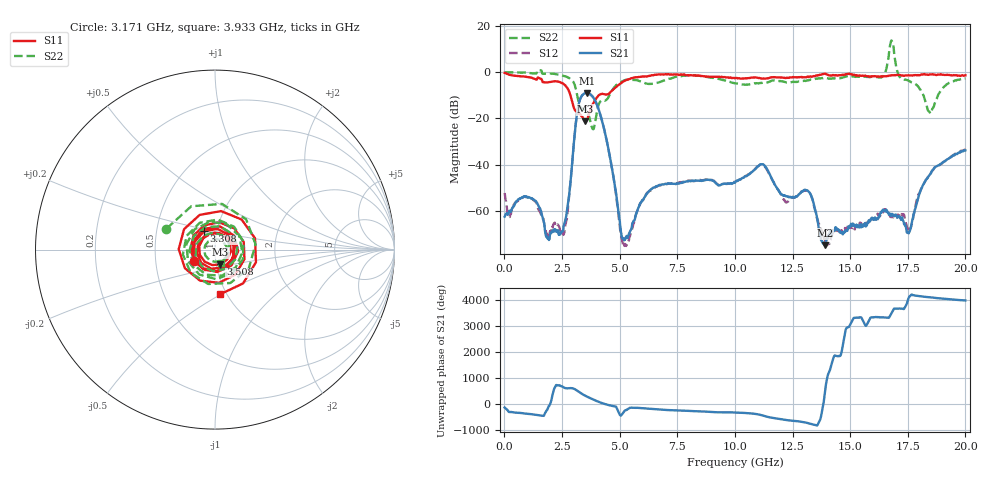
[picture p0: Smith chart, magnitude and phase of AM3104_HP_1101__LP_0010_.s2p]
!Created with skrf (http://scikit-rf.org).
# Hz S RI R 50.0
!freq ReS11 ImS11 ReS21 ImS21 ReS12 ImS12 ReS22 ImS22
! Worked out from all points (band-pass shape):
!   1601 points, 10 MHz to 20 GHz, reference 50 ohm
!   highest |S21| = -8.99 dB at 3.571 GHz (marker M1); lowest = -74.8 dB at 13.9 GHz (marker M2)
!   |S21| within 3 dB of the highest: 3.273 GHz to 3.92 GHz (647 MHz wide, 18 % of centre)
!   lowest |S11| = -21.2 dB at 3.508 GHz (marker M3), VSWR 1.19, Z = 52.4 - j8.66 ohm
!   |S11| at or under -10 dB: 2.866 GHz to 4.091 GHz (1.225 GHz wide, 35.2 % of centre)
!   |S22| runs from -24.6 to 13.7 dB; largest |S21 - S12| = 0.012
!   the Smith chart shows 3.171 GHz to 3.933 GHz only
!   S11 on the Smith chart (normalised r, x): 3.171 GHz: 0.78, -0.10; 3.308 GHz: 0.87, +0.18; 3.508 GHz: 1.05, -0.17; 3.933 GHz: 0.94, -0.50
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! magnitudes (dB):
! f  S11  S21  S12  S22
! 10 MHz  -0.3  -62.4  -52.2  0.0
! 972 MHz  -2.1  -53.8  -53.8  -0.2
! 1.872 GHz  -4.4  -71.8  -70.9  -0.7
! 2.534 GHz  -4.9  -68.5  -68.9  -1.5
! 3.171 GHz  -17.5  -16.7  -16.7  -10.6
! 3.308 GHz  -18.5  -11.1  -11.2  -15.3
! 3.346 GHz  -19.0  -10.4  -10.5  -15.7
! 3.508 GHz  -21.2  -9.1  -9.2  -16.5
! 3.571 GHz  -20.8  -9.0  -9.1  -17.3
! 3.933 GHz  -12.0  -12.2  -12.3  -21.9
! 5.182 GHz  -3.9  -72.4  -73.5  -3.7
! 6.682 GHz  -1.0  -49.0  -49.0  -4.5
! 10.01 GHz  -2.7  -47.7  -47.4  -4.8
! 11.19 GHz  -2.8  -39.8  -39.9  -4.6
! 12.19 GHz  -2.5  -53.3  -55.9  -4.3
! 13.34 GHz  -2.0  -54.2  -54.2  -3.3
! 13.9 GHz  -0.7  -74.8  -72.0  -2.4
! 16.35 GHz  -1.8  -60.5  -61.1  -2.3
! 16.68 GHz  -1.5  -61.4  -61.4  7.2
! 17.55 GHz  -1.4  -69.1  -69.1  -3.8
! 18.45 GHz  -1.0  -44.3  -44.3  -17.3
! 20 GHz  -1.4  -33.7  -33.4  -2.7
